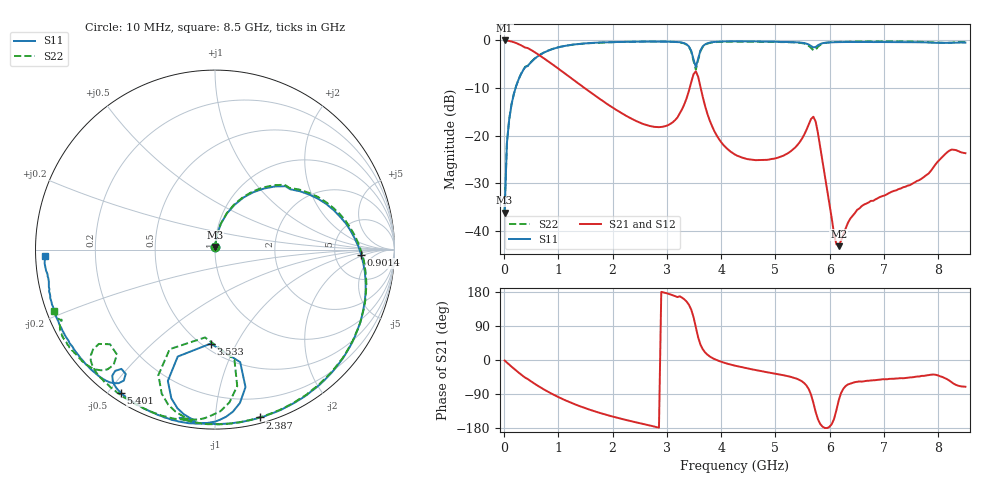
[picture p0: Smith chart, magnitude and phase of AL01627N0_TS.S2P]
!AVX CORPORATION
!PART NUMBER AL01627N0_TS
!DESCRIPTION: AIR CORE INDUCTOR, 27nH, 5 TURNS
!Agilent Technologies,E5071C,MY46102230,A.09.54
!Date: Mon Sep 03 16:35:17 2012
!Data & Calibration Information:
!Freq	S11:SOLT2(ON)	S21:SOLT2(ON)	S12:SOLT2(ON)	S22:SOLT2(ON)
# Hz S dB R 50
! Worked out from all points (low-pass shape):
!   201 points, 10 MHz to 8.5 GHz, reference 50 ohm
!   highest |S21| = -0.01 dB at 10 MHz (marker M1); lowest = -43.3 dB at 6.165 GHz (marker M2)
!   |S21| within 3 dB of the highest: start of sweep to 637.1 MHz
!   lowest |S11| = -36.3 dB at 10 MHz (marker M3), VSWR 1.03, Z = 50 + j1.54 ohm
!   |S11| at or under -10 dB: start of sweep to 212.4 MHz
!   |S22| runs from -36.0 to -0.2 dB; largest |S21 - S12| = 0.0025
!   S11 on the Smith chart (normalised r, x): 10 MHz: 1.00, +0.03; 901.5 MHz: 9.53, -1.70; 2.387 GHz: 0.04, -1.30; 3.533 GHz: 0.55, -0.79; 5.401 GHz: 0.03, -0.54; 8.5 GHz: 0.03, -0.02
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1e7  -36.26 88.6  -0.01 -1.3  -0.01 -1.2  -35.95 89.7
5.245e7  -21.61 82.7  -0.04 -6.8  -0.04 -6.9  -21.58 82.7
2.2225e8  -9.61 61.3  -0.55 -27.8  -0.53 -27.9  -9.59 61.9
5.194e8  -4.32 30.3  -2.15 -58.5  -2.14 -58.6  -4.29 31.3
9.0145e8  -1.77 -2.1  -5.11 -90.7  -5.10 -90.8  -1.76 -1.0
1.4533e9  -0.66 -36.2  -9.77 -124.9  -9.76 -125.0  -0.68 -35.9
2.3872e9  -0.28 -75.0  -16.70 -163.0  -16.70 -163.2  -0.29 -75.3
2.85415e9  -0.25 -89.8  -18.24 -178.5  -18.23 -178.7  -0.24 -89.9
3.19375e9  -0.38 -101.9  -16.22 166.0  -16.22 165.9  -0.35 -101.2
3.44845e9  -2.19 -109.7  -8.79 133.0  -8.79 133.0  -2.31 -114.3
3.53335e9  -5.61 -92.6  -6.49 86.3  -6.49 86.3  -6.15 -96.5
3.5758e9  -3.84 -77.4  -7.63 59.8  -7.63 59.8  -4.13 -80.0
3.70315e9  -0.83 -83.7  -13.77 20.2  -13.77 20.2  -0.90 -88.2
4.255e9  -0.19 -100.3  -24.01 -15.0  -24.00 -15.0  -0.27 -109.0
5.40115e9  -0.40 -123.3  -22.06 -49.8  -22.07 -49.8  -0.44 -134.6
5.6983e9  -1.47 -128.1  -16.04 -112.6  -16.04 -112.7  -2.08 -138.0
6.08035e9  -0.38 -133.0  -40.72 -155.3  -40.70 -154.9  -0.33 -138.3
6.16525e9  -0.36 -135.1  -43.28 -106.7  -43.52 -107.1  -0.29 -140.0
6.4624e9  -0.33 -141.3  -36.34 -58.5  -36.22 -59.6  -0.25 -143.6
7.09915e9  -0.34 -153.7  -32.07 -49.8  -32.09 -50.0  -0.19 -149.2
8.20285e9  -0.49 -172.2  -23.19 -54.2  -23.16 -54.3  -0.50 -155.4
8.5e9  -0.46 -177.8  -23.72 -70.5  -23.72 -70.2  -0.37 -159.2
